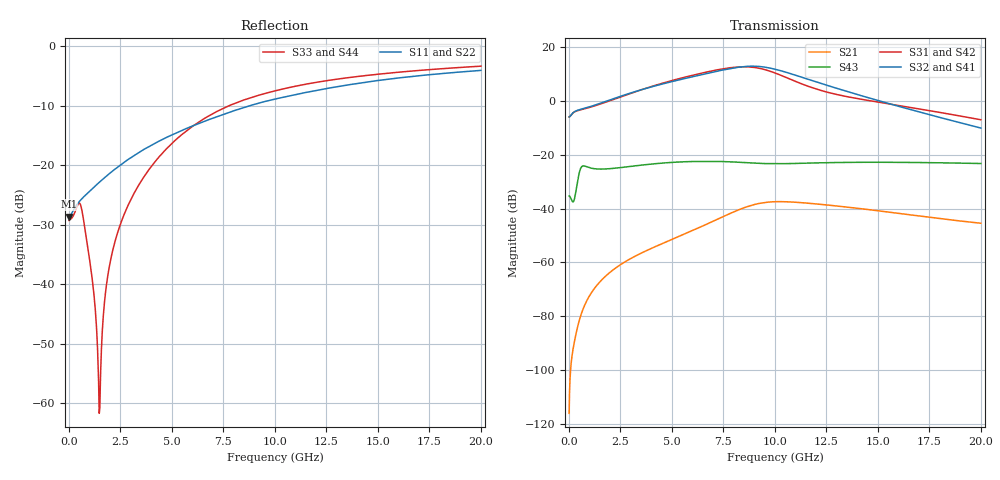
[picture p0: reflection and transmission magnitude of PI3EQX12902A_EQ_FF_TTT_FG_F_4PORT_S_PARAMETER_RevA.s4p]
! NPort=4 DATA=2000 NOISE=0 GROUPDELAY=0 COMPLEX_DATAFORMAT=POLAR
! NumOfBlock=1 NumOfParam=0
! .MODEL Smodel S TSTONEFILE=PI3EQX12902A_EQ_FF_TTT_FG_F_4PORT_S_PARAMETER_RevA.s4p TYPE=S
!  -- The above .MODEL line can be used for the S element in the netlist.
! The s parameter is extracted from the linear redriver, it is not bi-directional; only s(4,1)s(4,2) and s(3,1)s(3,2)
! should be the insertion loss
!Port definition:
!Port1 = input+
!Port2 = input-
!Port3 = output+
!Port4 = output-
# Hz S MA R  50
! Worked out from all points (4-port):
!   2000 points, 10 MHz to 20 GHz, reference 50 ohm
!   strongest paths, dB at 10 MHz, 5.01 GHz, 10.01 GHz, 15.01 GHz, 20 GHz:
!     S32: -6.0, 7.1, 11.7, 0.1, -10.2
!     S41: -6.0, 7.1, 11.6, 0.0, -10.1
!     S31: -6.0, 7.5, 10.3, -0.5, -7.1
!     S42: -6.0, 7.4, 10.1, -0.7, -7.2
!     S43: -35.3, -22.9, -23.4, -22.8, -23.3
!     S21: -116.0, -51.4, -37.5, -40.8, -45.5
!   lowest |S11| = -28.6 dB at 10 MHz (marker M1), VSWR 1.08, Z = 46.4 - j0.0607 ohm
!   |S11| at or under -10 dB: start of sweep to 8.781 GHz
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1e7  0.03704 -179.0  1.589e-06 51.9  0 0.0  0 0.0
     1.589e-06 51.9  0.03704 -179.0  0 0.0  0 0.0
     0.4992 1.1  0.4992 -178.9  0.03429 6.0  0.01709 -177.1
     0.4992 -178.9  0.4992 1.1  0.01709 -177.1  0.03429 6.0
5.84e9  0.2083 -112.0  0.003672 98.8  1.452e-06 -19.6  9.258e-07 89.6
        0.00367 98.8  0.2083 -112.0  9.279e-07 89.8  1.446e-06 -19.4
        2.861 -47.5  2.69 113.1  0.2024 -44.8  0.07377 146.4
        2.681 113.1  2.824 -48.0  0.07416 146.5  0.2018 -44.8
7.75e9  0.2769 -111.6  0.007865 79.8  6.076e-06 -76.7  3.891e-06 45.3
        0.00785 79.8  0.2768 -111.6  3.901e-06 45.3  6.048e-06 -76.3
        4.049 -101.1  3.893 58.9  0.3148 -63.9  0.07313 126.1
        3.869 58.8  3.983 -101.5  0.07361 126.0  0.3141 -63.8
9.15e9  0.3297 -113.2  0.01227 48.5  1.156e-05 -125.1  9.279e-06 -4.2
        0.01223 48.5  0.3296 -113.2  9.276e-06 -4.3  1.152e-05 -124.5
        4.057 -153.4  4.337 4.9  0.3843 -75.4  0.06853 115.1
        4.297 4.9  3.983 -153.8  0.06895 114.9  0.3839 -75.3
1.062e10  0.3795 -115.7  0.01335 11.8  1.499e-05 -164.9  1.451e-05 -61.2
          0.0133 12.0  0.3795 -115.7  1.446e-05 -61.3  1.5e-05 -164.1
          2.622 159.5  3.298 -50.6  0.4462 -85.1  0.06779 107.9
          3.261 -50.3  2.564 159.3  0.06805 107.6  0.4462 -85.0
1.299e10  0.4561 -119.5  0.01116 -26.5  2.231e-05 155.3  1.85e-05 -130.8
          0.01115 -26.2  0.4562 -119.5  1.836e-05 -130.7  2.25e-05 156.0
          1.306 124.6  1.701 -112.1  0.5273 -97.4  0.0713 92.5
          1.685 -111.4  1.273 124.9  0.07128 92.2  0.5277 -97.4
2e10  0.626 -131.7  0.005272 -75.3  4.094e-05 50.8  1.791e-05 98.1
      0.00533 -75.3  0.626 -131.7  1.771e-05 99.0  4.141e-05 50.9
      0.4429 38.0  0.3105 131.6  0.6794 -119.6  0.06843 46.2
      0.3115 132.6  0.438 38.8  0.06833 46.1  0.6797 -119.6
